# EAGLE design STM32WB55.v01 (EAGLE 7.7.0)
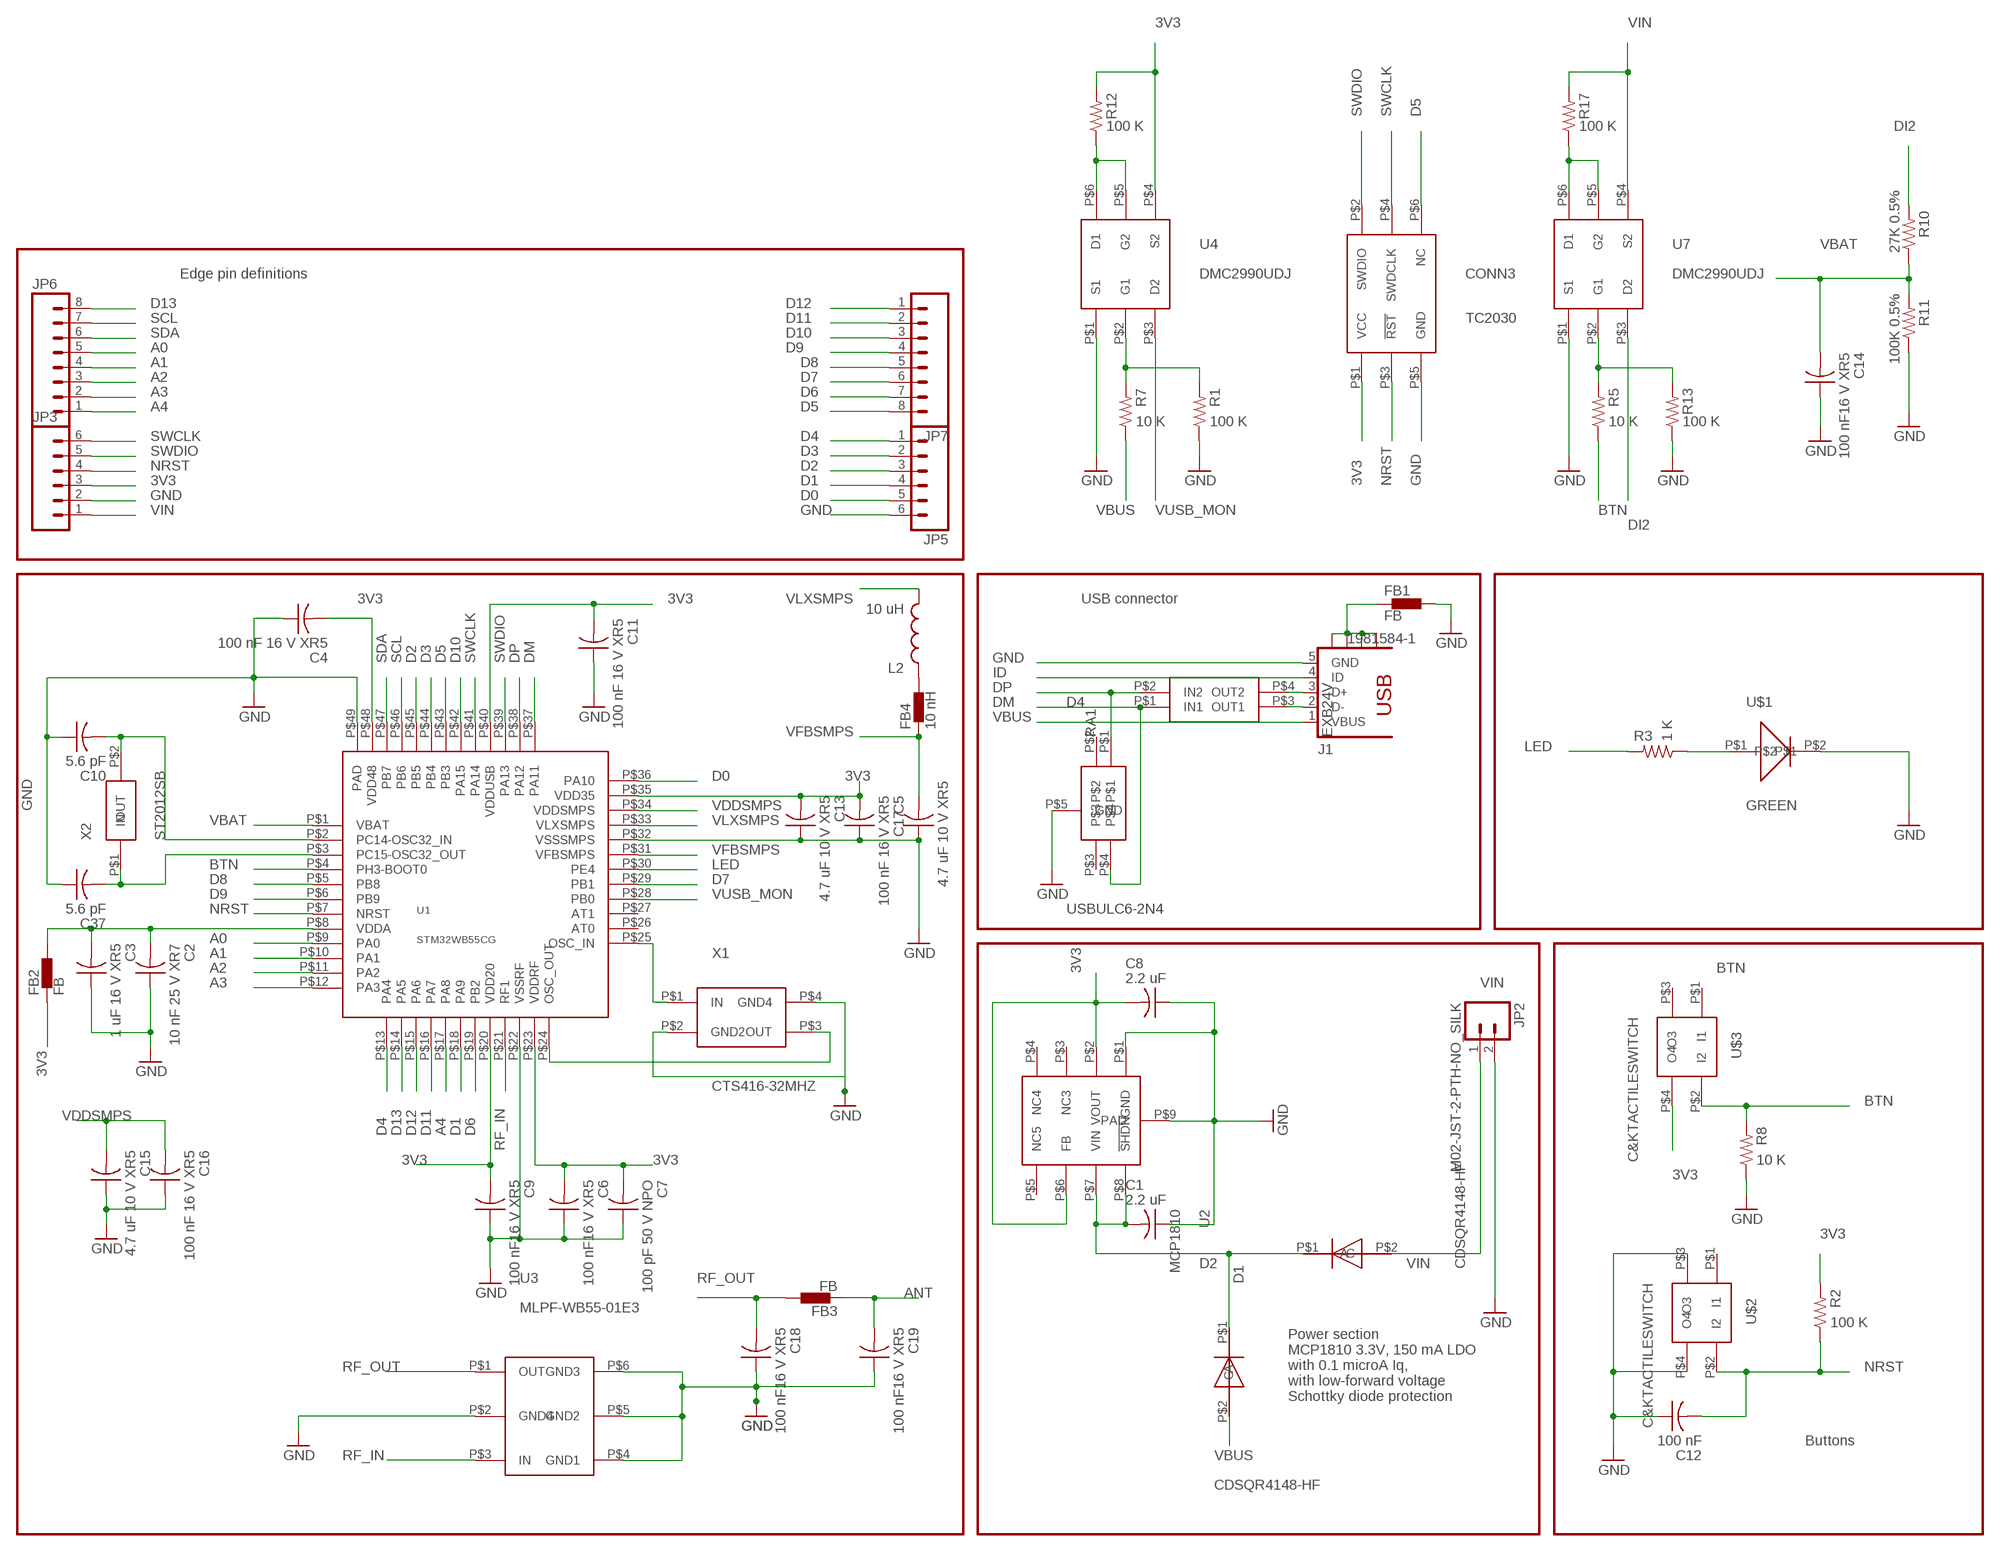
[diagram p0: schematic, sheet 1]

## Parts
C1  2.2 uF  C-US  [C0402_B]
C2  10 nF 25 V XR7  C-US  [C0402_B]
C3  1 uF 16 V XR5  C-US  [C0402_B]
C4  100 nF 16 V XR5  C-US  [C0402_B]
C5  100 nF 16 V XR5  C-US  [C0402_B]
C6  100 nF16 V XR5  C-US  [C0402_B]
C7  100 pF 50 V NPO  C-US  [C0402_B]
C8  2.2 uF  C-US  [C0402_B]
C9  100 nF16 V XR5  C-US  [C0402_B]
C10  5.6 pF  C-US  [C0402_B]
C11  100 nF 16 V XR5  C-US  [C0402_B]
C12  100 nF  C-US  [C0402_B]
C13  4.7 uF 10 V XR5  C-US  [C0402_B]
C14  100 nF16 V XR5  C-US  [C0402_B]
C15  4.7 uF 10 V XR5  C-US  [C0402_B]
C16  100 nF 16 V XR5  C-US  [C0402_B]
C17  4.7 uF 10 V XR5  C-US  [C0402_B]
C18  100 nF16 V XR5  C-US  [C0402_B]
C19  100 nF16 V XR5  C-US  [C0402_B]
C37  5.6 pF  C-US  [C0402_B]
CONN3  TC2030  [TC2030]
D1  CDSQR4148-HF  [CDSQR4148-HF]
D2  CDSQR4148-HF  [CDSQR4148-HF]
D4  USBULC6-2N4  [USBULC6-2N4]
FB1  FB  BLM15H  [0402]
FB2  FB  BLM15H  [0402]
FB3  FB  BLM15H  [0402]
FB4  10 nH  BLM15H  [0402]
J1  1981584-1  [1981584-1]
JP2  M02-JST-2-PTH-NO_SILK  [JST-2-PTH-NS]
JP3  M06NO_SILK  [1X06_NO_SILK]
JP5  M06NO_SILK  [1X06_NO_SILK]
JP6  M08NO_SILK  [1X08_NO_SILK]
JP7  M08NO_SILK  [1X08_NO_SILK]
L2  10 uH  INDUCTOR0805  [0805]
R1  100 K  R-US_  [R0402_B]
R2  100 K  R-US_  [R0402_B]
R3  1 K  R-US_  [R0402_B]
R5  10 K  R-US_  [R0402_B]
R7  10 K  R-US_  [R0402_B]
R8  10 K  R-US_  [R0402_B]
R10  27K 0.5%  R-US_  [R0402_B]
R11  100K 0.5%  R-US_  [R0402_B]
R12  100 K  R-US_  [R0402_B]
R13  100 K  R-US_  [R0402_B]
R17  100 K  R-US_  [R0402_B]
RA1  EXB24V  [EXB24V]
U1  STM32WB55CG  [ST32WB55CG]
U2  MCP1810  [MCP1810]
U3  MLPF-WB55-01E3  [MLPF-WB55-01E3]
U4  DMC2990UDJ  [DMC2990UDJ]
U7  DMC2990UDJ  [DMC2990UDJ]
U$1  GREEN  0402LED  [0402LED]
U$2  C&KTACTILESWITCH  [C&KTACTILESWITCH]
U$3  C&KTACTILESWITCH  [C&KTACTILESWITCH]
X1  CTS416-32MHZ  [CTS416-32MHZ]
X2  ST2012SB  [ST2012SB]

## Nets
3V3: C4.2 C5.2 C6.2 C7.2 C8.2 C9.2 C11.2 C13.2 CONN3.P$1(VCC) FB2.1 JP3.3 R2.2 R12.2 U1.P$20(VDD20) U1.P$23(VDDRF) U1.P$35(VDD35) U1.P$40(VDDUSB) U1.P$48(VDD48) U2.P$2(VOUT) U2.P$6(FB) U4.P$4(S2) U$3.P$4(O4)
A0: JP6.5 U1.P$9(PA0)
A1: JP6.4 U1.P$10(PA1)
A2: JP6.3 U1.P$11(PA2)
A3: JP6.2 U1.P$12(PA3)
A4: JP6.1 U1.P$17(PA8)
ANT: C19.2 FB3.1
BTN: R5.1 R8.2 U1.P$4(PH3-BOOT0) U$3.P$2(I2)
D0: JP5.5 U1.P$36(PA10)
D1: JP5.4 U1.P$18(PA9)
D2: JP5.3 U1.P$45(PB5)
D3: JP5.2 U1.P$44(PB4)
D4: JP5.1 U1.P$13(PA4)
D5: CONN3.P$6(NC) JP7.8 U1.P$43(PB3)
D6: JP7.7 U1.P$19(PB2)
D7: JP7.6 U1.P$29(PB1)
D8: JP7.5 U1.P$5(PB8)
D9: JP7.4 U1.P$6(PB9)
D10: JP7.3 U1.P$42(PA15)
D11: JP7.2 U1.P$16(PA7)
D12: JP7.1 U1.P$15(PA6)
D13: JP6.8 U1.P$14(PA5)
DI2: R10.2 U7.P$3(D2)
DM: D4.P$4 RA1.P$1(IN1) U1.P$37(PA11)
DP: D4.P$1 RA1.P$2(IN2) U1.P$38(PA12)
GND: C1.1 C2.1 C3.1 C4.1 C5.1 C6.1 C7.1 C8.1 C9.1 C10.1 C11.1 C12.1 C13.1 C14.1 C15.1 C16.1 C17.1 C18.1 C19.1 C37.1 CONN3.P$5(GND) D4.P$5(GND) FB1.2 J1.5(GND) JP2.2 JP3.2 JP5.6 R1.1 R8.1 R11.1 R13.1 U1.P$22(VSSRF) U1.P$32(VSSSMPS) U1.P$49(PAD) U2.P$1(GND) U2.P$9(PAD) U3.P$2(GND4) U3.P$4(GND1) U3.P$5(GND2) U3.P$6(GND3) U4.P$1(S1) U7.P$1(S1) U$1.P$2 U$2.P$3(O3) U$2.P$4(O4) X1.P$2(GND2) X1.P$4(GND4)
ID: J1.4(ID)
LED: R3.2 U1.P$30(PE4)
N$1: R3.1 U$1.P$1
N$2: C2.2 C3.2 FB2.2 U1.P$8(VDDA)
N$3: U1.P$25(OSC_IN) X1.P$1(IN)
N$4: U1.P$24(OSC_OUT) X1.P$3(OUT)
N$5: FB4.2 L2.1
N$7: C10.2 U1.P$2(PC14-OSC32_IN) X2.P$2(OUT)
N$8: C37.2 U1.P$3(PC15-OSC32_OUT) X2.P$1(IN)
N$10: R1.2 R7.2 U4.P$2(G1)
N$11: R12.1 U4.P$5(G2) U4.P$6(D1)
N$12: R5.2 R13.2 U7.P$2(G1)
N$13: R17.1 U7.P$5(G2) U7.P$6(D1)
N$31: J1.3(D+) RA1.P$4(OUT2)
N$33: J1.2(D-) RA1.P$3(OUT1)
NRST: C12.2 CONN3.P$3(!RST) JP3.4 R2.1 U1.P$7(NRST) U$2.P$2(I2)
PWRIN: C1.2 D1.P$1(C) D2.P$1(C) U2.P$7(VIN) U2.P$8(!SHDN)
RF_IN: U1.P$21(RF1) U3.P$3(IN)
RF_OUT: C18.2 FB3.2 U3.P$1(OUT)
SCL: JP6.7 U1.P$46(PB6)
SDA: JP6.6 U1.P$47(PB7)
SWCLK: CONN3.P$4(SWDCLK) JP3.6 U1.P$41(PA14)
SWDIO: CONN3.P$2(SWDIO) JP3.5 U1.P$39(PA13)
USB_SHIELD: FB1.1 J1.S1 J1.S2 J1.S3 J1.S4
VBAT: C14.2 R10.1 R11.2 U1.P$1(VBAT)
VBUS: D2.P$2(A) J1.1(VBUS) R7.1
VDDSMPS: C15.2 C16.2 U1.P$34(VDDSMPS)
VFBSMPS: C17.2 FB4.1 U1.P$31(VFBSMPS)
VIN: D1.P$2(A) JP2.1 JP3.1 R17.2 U7.P$4(S2)
VLXSMPS: L2.2 U1.P$33(VLXSMPS)
VUSB_MON: U1.P$28(PB0) U4.P$3(D2)
Unconnected: D4.P$2 D4.P$3 U1.P$26(AT0) U1.P$27(AT1) U2.P$3(NC3) U2.P$4(NC4) U2.P$5(NC5) U$2.P$1(I1) U$3.P$1(I1) U$3.P$3(O3)

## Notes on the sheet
- Edge pin definitions
- USB connector
- Power section
  MCP1810 3.3V, 150 mA LDO
  with 0.1 microA Iq, 
  with low-forward voltage 
  Schottky diode protection
- Buttons

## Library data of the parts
C1-C19 C37 = Spark:C-US: Capacitor
CONN3 = Kris:TC2030: TC2030 SWD pogo pin contact pad
D1 D2 = Kris:CDSQR4148-HF: ComChip's CDSQR4148-HF high speed 150 mA Io diode
D4 = Kris:USBULC6-2N4: ST TVS diode ESD Protection USBULC6-2N4
FB1-FB4 = STM32L433SARA.AssetTracker.v01:BLM15H: EMIFIL (R) Chip Ferrite Bead for GHz Noise
J1 = con-usb:1981584-1: Receptacle, micro-USB, type A/B Tyco Electronics; MF: Hirose; MPN: ZX62-AB-5PA(11)
JP2 = SparkFun-Connectors:M02: Standard 2-pin 0.1" header. Use with
JP3 JP5 = SparkFun-Connectors:M06: Header 6 Standard 6-pin 0.1" header. Use with straight break away headers (SKU : PRT-00116), right angle break away headers (PRT-00553), swiss pins (PRT-00743), machine pins (PRT-00117), and female headers (PRT-00115). Molex polarized connector foot print use with SKU : PRT-08094 with associated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
JP6 JP7 = SparkFun-Connectors:M08: Header 8 Standard 8-pin 0.1" header. Use with straight break away headers (SKU : PRT-00116), right angle break away headers (PRT-00553), swiss pins (PRT-00743), machine pins (PRT-00117), and female headers (PRT-00115).
L2 = SparkFun-Passives:INDUCTOR: Inductors
R1-R3 R5 R7 R8 R10-R13 R17 = Spark:R-US_: 0402 Resistor
RA1 = Kris:EXB24V: Panasonic EXB24 22 Ohm series resistor pair
U1 = Kris:STM32WB55CG: STM32WB55CG 7 mm x 7 mm UFQFPN48 https://www.st.com/en/microcontrollers/stm32wbx5.html?querycriteria=productId=LN2047
U2 = Kris:MCP1810: MCP1810 3.0 V Low Iq LDO http://ww1.microchip.com/downloads/en/DeviceDoc/20005623A.pdf
U3 = Kris:MLPF-WB55-01E3: MLPF-WB55-01E3
U4 U7 = Kris:DMC2990UDJ: DMC2990UDJ dual N-Type and P-Type MOSFET COMPLEMENTARY PAIR ENHANCEMENT MODE MOSFET https://www.diodes.com/assets/Datasheets/DMC2990UDJ.pdf
U$1 = Kris:0402LED: 0402led
U$2 U$3 = Kris:C&KTACTILESWITCH: C&K Tactile Switch 611-PTS810SJS250SMTR
X1 = Kris:CTS416-32MHZ: 32 MHz CTS416 crystal
X2 = Kris:ST2012SB: Kyocera 2.0 x 1.2 mm 32.768 20kHz ppm 4 pf crystal

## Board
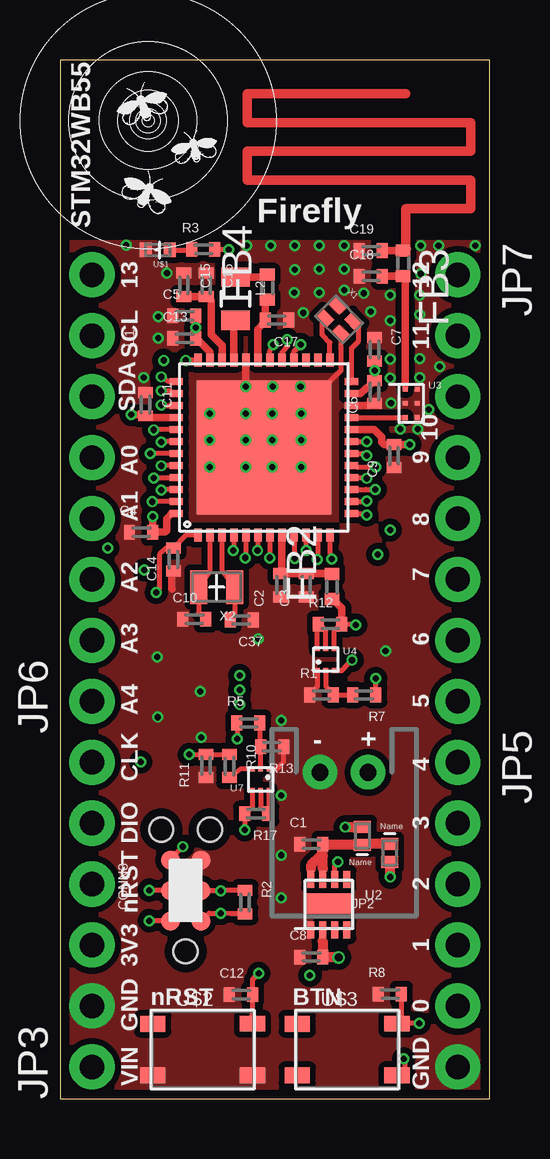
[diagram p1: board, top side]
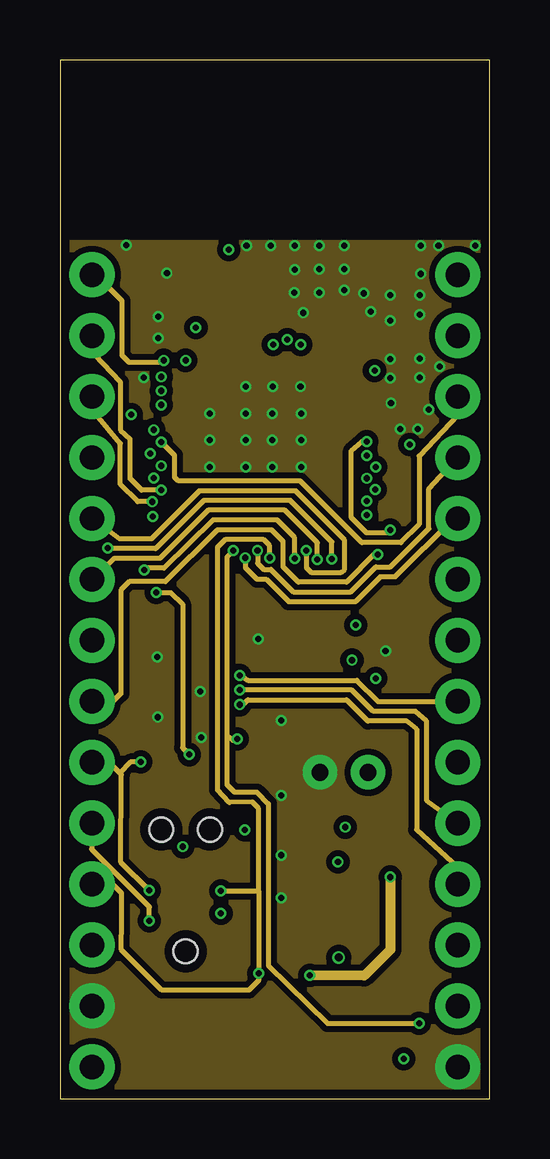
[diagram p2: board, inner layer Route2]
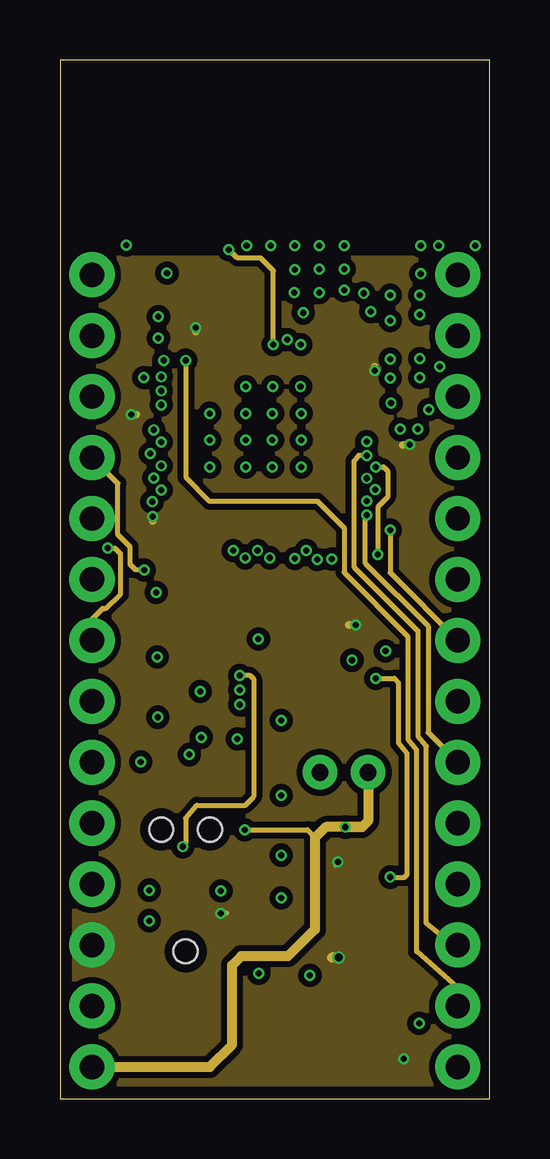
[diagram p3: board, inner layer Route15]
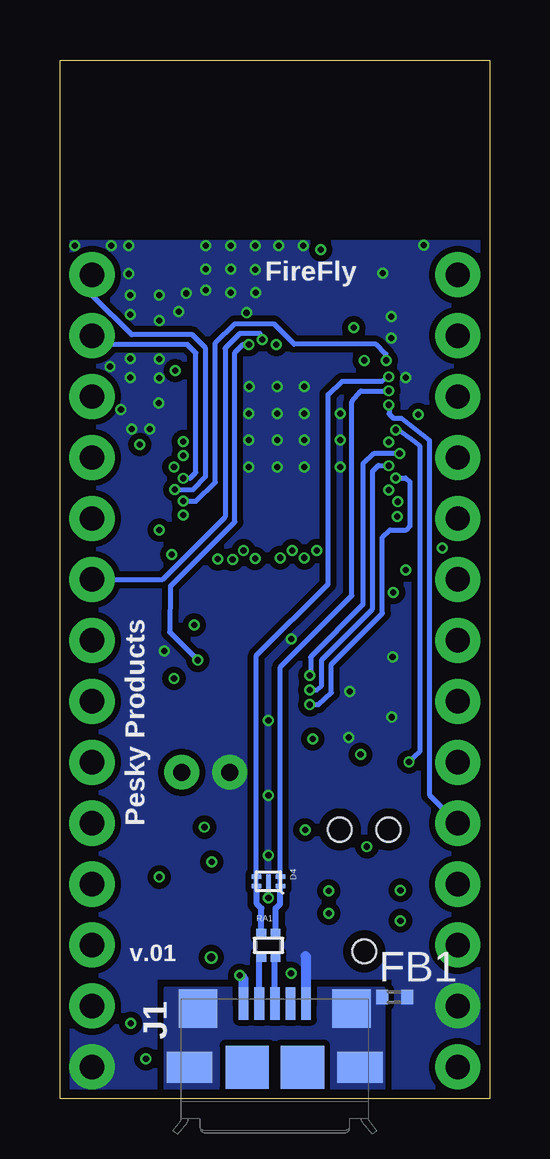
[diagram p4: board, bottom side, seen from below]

Size 17.91 x 43.31 mm. Coordinates in mm from the lower left corner, seen from the top.
Outline: 0,0 17.91,0 17.91,43.31 0,43.31 0,0
Copper layers (1*2*15*16): Top 0.035559375mm / dielectric 0.17018125mm / Route2 0.01778125mm / dielectric 47mil / Route15 0.01778125mm / dielectric 0.17018125mm / Bottom 0.035559375mm
Design rules "OSHPark-4layer *": minimum track width 5mil, minimum drill 10mil, track to track 5mil, track to pad 5mil, pad to pad 5mil, via to via 5mil, smd to smd 5mil, copper to edge 15mil, drill to drill 6mil, minimum pad ring 4mil, minimum via ring 4mil, stop-mask expansion 4mil, vias tented up to drill 20mil, thermal gap 10mil

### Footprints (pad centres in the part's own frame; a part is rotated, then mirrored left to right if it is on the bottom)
C0402_B = smd 0.457 x 0.61: 1 -0.483,0; 2 0.483,0
TC2030 = smd 0.787 x 0.787: P$1 -1.27,-0.635; P$2 -1.27,0.635; P$3 0,-0.635; P$4 0,0.635; P$5 1.27,-0.635; P$6 1.27,0.635 | hole 0.991: -2.54,0; 2.54,1.016; 2.54,-1.016
CDSQR4148-HF = smd 0.7 x 0.5: P$1 0,0.375; P$2 0,-0.375
USBULC6-2N4 = smd 0.2 x 0.4: P$1 0.2,0.5; P$2 -0.2,0.5; P$3 -0.2,-0.5; P$4 0.2,-0.5 | smd 0.6 x 0.2: P$5 0,0
0402 = smd 0.5 x 0.61: 1 -0.5,0; 2 0.55,0
1981584-1 = smd 0.4 x 1.35: 1 -1.3,4.1; 2 -0.65,4.1; 3 0,4.1; 4 0.65,4.1; 5 1.3,4.1 | smd 1.8 x 1.8: M1 -1.15,1.45; M2 1.15,1.45 | smd 1.9 x 1.3: S1 -3.55,1.45; S2 3.55,1.45 | smd 1.6 x 1.6: S3 -3.2,3.885; S4 3.2,3.885
JST-2-PTH-NS = drill 0.7 pad 1.448: 1 -1,0; 2 1,0
1X06_NO_SILK = drill 1.016 pad 1.88: 1 0,0; 2 2.54,0; 3 5.08,0; 4 7.62,0; 5 10.16,0; 6 12.7,0
1X08_NO_SILK = drill 1.016 pad 1.88: 1 0,0; 2 2.54,0; 3 5.08,0; 4 7.62,0; 5 10.16,0; 6 12.7,0; 7 15.24,0; 8 17.78,0
0805 = smd 0.8 x 1.2: 1 -0.9,0; 2 0.9,0
R0402_B = smd 0.457 x 0.61: 1 -0.483,0; 2 0.483,0
EXB24V = smd 0.4 x 0.36: P$1 -0.3,0.5; P$2 0.3,0.5; P$3 -0.3,-0.5; P$4 0.3,-0.5
ST32WB55CG = smd 0.55 x 0.3: P$1 -3.65,2.75; P$2 -3.65,2.25; P$3 -3.65,1.75; P$4 -3.65,1.25; P$5 -3.65,0.75; P$6 -3.65,0.25; P$7 -3.65,-0.25; P$8 -3.65,-0.75; P$9 -3.65,-1.25; P$10 -3.65,-1.75; P$11 -3.65,-2.25; P$12 -3.65,-2.75; P$25 3.65,-2.75; P$26 3.65,-2.25; P$27 3.65,-1.75; P$28 3.65,-1.25; P$29 3.65,-0.75; P$30 3.65,-0.25; P$31 3.65,0.25; P$32 3.65,0.75; P$33 3.65,1.25; P$34 3.65,1.75; P$35 3.65,2.25; P$36 3.65,2.75 | smd 0.3 x 0.55: P$13 -2.75,-3.65; P$14 -2.25,-3.65; P$15 -1.75,-3.65; P$16 -1.25,-3.65; P$17 -0.75,-3.65; P$18 -0.25,-3.65; P$19 0.25,-3.65; P$20 0.75,-3.65; P$21 1.25,-3.65; P$22 1.75,-3.65; P$23 2.25,-3.65; P$24 2.75,-3.65; P$37 2.75,3.65; P$38 2.25,3.65; P$39 1.75,3.65; P$40 1.25,3.65; P$41 0.75,3.65; P$42 0.25,3.65; P$43 -0.25,3.65; P$44 -0.75,3.65; P$45 -1.25,3.65; P$46 -1.75,3.65; P$47 -2.25,3.65; P$48 -2.75,3.65 | smd 5.6 x 5.6: P$49 0,0
MCP1810 = smd 0.3 x 0.7: P$1 -0.75,-1.05; P$2 -0.25,-1.05; P$3 0.25,-1.05; P$4 0.75,-1.05; P$5 0.75,1.05; P$6 0.25,1.05; P$7 -0.25,1.05; P$8 -0.75,1.05 | smd 1.95 x 0.95: P$9 0,0
MLPF-WB55-01E3 = smd 0.2 x 0.2: P$1 -0.25,0.587; P$2 -0.25,0; P$3 -0.25,-0.587; P$4 0.25,-0.587; P$5 0.25,0; P$6 0.25,0.587
DMC2990UDJ = smd 0.2 x 0.2: P$1 -0.35,-0.45; P$2 0,-0.45; P$3 0.35,-0.45; P$4 0.35,0.45; P$5 0,0.45; P$6 -0.35,0.45
0402LED = smd 0.5 x 0.6: P$1 -0.5,0; P$2 0.5,0
C&KTACTILESWITCH = smd 1.05 x 0.65: P$1 -2.075,1.073; P$2 2.075,1.075; P$3 -2.075,-1.075; P$4 2.075,-1.075
CTS416-32MHZ = smd 0.67 x 0.48: P$1 -0.485,-0.38; P$2 0.485,-0.38; P$3 0.485,0.38; P$4 -0.485,0.38
ST2012SB = smd 0.7 x 1.4: P$1 -0.75,0; P$2 0.75,0

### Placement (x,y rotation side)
C1  10.46,10.62 0 top
C2  9.19,21.41 90 top
C3  10.26,21.41 90 top
C4  3.38,23.62 0 top
C5  5.18,32.64 0 top
C6  13.11,29.46 90 top
C7  13.11,31.24 270 top
C8  10.46,5.92 0 top
C9  13.92,26.8 90 top
C10  5.59,19.99 0 top
C11  3.56,28.96 270 top
C12  7.54,4.34 0 top
C13  5.18,31.7 0 top
C14  4.72,22.48 90 top
C15  5.16,33.93 270 top
C16  6.1,33.93 270 top
C17  9.04,32.46 180 top
C18  12.95,34.29 0 top
C19  12.95,35.36 0 top
C37  7.57,19.96 180 top
CONN3  5.23,8.69 90 top
D1  12.6,10.97 180 top
D2  13.74,10.26 0 top
D4  9.22,9.07 270 bottom
FB1  3.99,4.24 0 bottom
FB2  11.33,21.34 90 top
FB3  14.3,34.85 270 top
FB4  8.64,33.81 90 top
J1  8.95,-0.13 0 bottom
JP2  11.84,13.61 180 top
JP3  1.33,1.33 90 top
JP5  16.57,14.03 270 top
JP6  1.33,16.57 90 top
JP7  16.57,34.35 270 top
L2  7.32,33.35 270 top
R1  10.9,16.84 0 top
R2  7.71,8.2 270 top
R3  5.97,35.41 0 top
R5  7.85,15.67 0 top
R7  12.67,16.84 180 top
R8  13.74,4.37 0 top
R10  7.06,13.88 270 top
R11  6.08,13.88 90 top
R12  11.25,19.79 0 top
R13  8.84,14.68 180 top
R17  8.18,11.89 180 top
RA1  9.22,6.4 0 bottom
U1  8.5,27.15 90 top
U2  11.2,8.1 0 top
U3  14.63,28.99 0 top
U4  11.07,18.31 0 top
U7  8.36,13.31 180 top
U$1  4.06,35.38 180 top
U$2  5.94,2.06 0 top
U$3  11.96,2.06 0 top
X1  11.63,32.49 315 top
X2  6.53,21.34 180 top

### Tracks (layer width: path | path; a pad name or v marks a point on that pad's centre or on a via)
3V3  (via drill 0.25, 0.33)
  Top 0.203: U2.P$6 11.45,9.72 v11.58,9.88 | U$3.P$4 14.38,1.22 14.38,1.63 v14.33,1.68 | U4.P$4 11.42,19.58 R12.2 12.27,19.79 v12.32,19.76 | CONN3.P$1 6.21,7.73 v6.71,7.73 7.1,7.72 R2.2
  Top 0.305: U1.P$35 6.25,31.14 5.69,31.7 5.69,31.67 C13.2 v5.66,32.16 C5.2 | U1.P$40 3.54,28.4 3.53,28.4 3.45,28.4 | C7.2 v13.11,30.35 C6.2 12.51,29.4 U1.P$23 | 10.95,5.87 C8.2 | U2.P$2 10.95,6.58 | v3.86,24.28 C4.2 4.37,23.62 4.45,23.7 4.45,24.18 4.64,24.4 U1.P$48 | v14.58,27.28 C9.2 13.51,27.28 13.41,27.38 13.41,27.58 13.09,27.9 U1.P$20 | 3.45,28.4 C11.2 3.33,28.5 v2.97,28.52 | 3.45,28.4 3.45,28.42 | FB2.1 11.37,20.84 11.73,20.47 R12.2
  Top 0.406: v11.61,5.89 11.53,5.92 C8.2 10.95,6.58
  Route15 0.203: v11.58,9.88 11.48,9.75 | v14.33,1.68 14.33,1.63 14.38,1.57 | v6.71,7.73 6.95,7.73
  Route15 0.305: v5.66,32.16 5.66,31.98 | v12.32,19.76 12.04,19.76 | v2.97,28.52 3.17,28.52 | v13.11,30.35 13.11,30.53 | v3.86,24.28 3.86,24.08 | v14.58,27.28 14.28,27.25
  Route15 0.406: v11.61,5.89 11.33,5.89
  pour Route15 (isolate 0.254, no thermals): 0.64,35.05 17.27,35.05 17.27,0.64 0.64,0.64
A0  (via drill 0.25)
  Top 0.203: v9.78,22.53 9.78,23.41 U1.P$9
  Route2 0.203: v9.78,22.53 9.78,23.39 9.04,24.13 6.38,24.13 4.34,22.12 3.5,22.12 v3.5,22.05
  Route15 0.203: v3.5,22.05 3.15,22.05 2.92,22.28 2.92,23.01 2.41,23.52 2.41,25.65 JP6.5
A1  (via drill 0.25)
  Top 0.203: U1.P$10 10.25,22.88 v10.26,22.86
  Route2 0.203: JP6.4 2.49,23.34 3.81,23.34 5.82,25.35 9.8,25.35 11.86,23.29 11.86,22.07 11.71,21.95 10.46,21.95 10.26,22.15 v10.26,22.86
A2  (via drill 0.25)
  Top 0.203: U1.P$11 10.75,22.58 v10.72,22.48
  Route2 0.203: v10.72,22.48 10.72,23.19 9.37,24.54 6.17,24.54 4.17,22.53 2.26,22.53 JP6.3
A3  (via drill 0.25)
  Top 0.203: U1.P$12 11.25,22.69 v11.33,22.5
  Route2 0.203: v11.33,22.5 11.33,23.22 9.6,24.94 5.99,24.94 3.99,22.94 2.08,22.94 v1.98,22.96
  Route15 0.203: v1.98,22.96 2.29,22.96 2.52,22.73 2.52,21.03 1.91,20.45 1.78,20.45 1.33,20 JP6.2
A4  (via drill 0.25)
  Top 0.203: U1.P$17 12.33,26.4 12.37,26.34 v13.16,26.34
  Route2 0.203: JP6.1 1.35,16.59 2.21,16.59 2.54,16.89 2.54,21.21 2.9,21.57 4.39,21.57 6.55,23.72 8.81,23.72 9.3,23.24 9.3,22.17 9.93,21.54 11.94,21.54 13.08,22.68 v13.25,22.7
  Route15 0.203: v13.25,22.7 13.25,24.66 13.65,25.09 13.65,26.18 13.49,26.34 v13.16,26.34
ANT
  Top 0.305: C19.2 14.22,35.36 FB3.1
  Top 0.4: 14.41,35.43 14.41,37.1 17.11,37.1 17.11,38.3 7.81,38.3 7.81,39.5 17.11,39.5 17.11,40.7 7.81,40.7 7.81,41.9 14.41,41.9
  Top 0.406: FB3.1 14.32,35.35 14.41,35.43
BTN  (via drill 0.25)
  Top 0.203: U1.P$4 7.25,22.94 v7.21,22.86 | v14.96,3.15 13.98,3.15 U$3.P$2 14.22,3.39 R8.2 | R5.1 v7.38,15
  Route2 0.203: v14.96,3.15 11.15,3.15 8.69,5.56 8.69,12.31 8.22,12.78 7.28,12.78 6.96,13.09 6.96,15.14 | 6.96,15.14 6.96,22.58 v7.21,22.86 | v7.38,15 7.19,14.95 6.96,15.14
D0  (via drill 0.25)
  Top 0.203: U1.P$36 5.33,30.8 v5.23,30.79
  Route15 0.203: JP5.5 16.57,4.64 14.86,6.15 14.86,14.55 14.5,14.99 14.5,19.25 11.84,21.95 11.84,23.8 10.72,24.92 6.22,24.92 5.26,25.91 5.26,30.76 v5.23,30.79
D1  (via drill 0.25)
  Top 0.203: U1.P$18 12.62,26.9 v12.78,26.81
  Route15 0.203: JP5.4 16.34,6.41 15.27,7.32 15.27,14.71 14.91,15.14 14.91,19.51 12.24,22.17 12.24,26.59 12.45,26.82 v12.78,26.81
D2  (via drill 0.25)
  Top 0.203: U1.P$45 4.7,25.9 4.67,25.93 4.7,25.93 4.62,25.88 v3.91,25.88
  Route2 0.203: JP5.3 16.59,8.97 16.59,9.65 14.86,11.23 14.86,15.42 14.45,15.75 12.83,15.75 11.94,16.64 7.82,16.64 7.64,16.43 v7.49,16.43
  Bottom 0.203: v3.91,25.88 3.5,25.88 3.33,25.73 3.33,23.88 3.48,23.72 4.17,23.72 4.47,23.42 4.47,20.24 6.6,18.11 6.6,16.94 7.14,16.43 v7.49,16.43
D3  (via drill 0.25)
  Top 0.203: U1.P$44 4.25,26.4 v4.22,26.39
  Route2 0.203: v7.49,17.04 12.17,17.04 13.06,16.15 14.81,16.15 15.27,15.75 15.27,12.45 JP5.2
  Bottom 0.203: v4.22,26.39 4.31,26.4 4.64,26.4 4.88,26.17 4.88,20.42 7.01,18.29 7.01,17.22 7.21,17.04 v7.49,17.04
D4  (via drill 0.25)
  Top 0.203: U1.P$13 12.68,24.4 v12.78,24.33
  Route15 0.203: JP5.1 15.34,15.27 15.34,19.71 12.72,22.33 12.72,24.16 v12.78,24.33
D5  (via drill 0.25)
  Top 0.203: U1.P$43 v3.76,26.9 | CONN3.P$6 4.6,10.03 v5.12,10.52
  Route2 0.203: JP7.8 13.26,16.56 12.37,17.45 7.82,17.45 7.57,17.65 v7.49,17.65
  Route15 0.203: 7.48,17.67 7.52,17.67 | 7.52,17.67 7.9,17.67 8.06,17.5 8.06,12.6 7.71,12.24 5.7,12.24 5.23,11.7 5.23,10.63 v5.12,10.52 | v7.49,17.65 7.51,17.65 7.52,17.67
  Bottom 0.203: v3.76,26.9 4.83,26.9 5.28,26.47 5.28,20.6 7.47,18.41 7.47,17.7 v7.49,17.65
D6  (via drill 0.25)
  Top 0.203: U1.P$19 12.72,27.4 v12.78,27.39
  Route2 0.203: v13.77,23.71 13.6,23.6 12.78,23.6 12.14,24.23 12.14,27.03 12.57,27.41 12.76,27.41 v12.78,27.39
  Route15 0.203: v13.77,23.71 13.75,21.93 JP7.7
D7  (via drill 0.25)
  Top 0.203: U1.P$29 9.25,31.09 9.47,31.37 v9.47,31.65
  Bottom 0.203: v9.47,31.65 9.47,31.77 9.58,31.9 10.41,31.9 11.02,31.29 11.02,24.26 13.63,21.65 JP7.6
D8  (via drill 0.25)
  Top 0.203: U1.P$5 7.75,22.61 v7.72,22.55
  Route2 0.203: v7.72,22.55 7.72,22.15 8.2,21.67 8.59,21.67 9.53,20.73 12.32,20.73 13.36,21.77 13.97,21.77 16.38,24.18 JP7.5
D9  (via drill 0.25)
  Top 0.203: U1.P$6 8.25,22.98 v8.23,22.86
  Route2 0.203: JP7.4 15.37,25.43 15.37,23.77 13.77,22.17 13.16,22.17 12.12,21.13 9.73,21.13 8.79,22.07 8.48,22.07 8.23,22.33 v8.23,22.86
D10  (via drill 0.25)
  Top 0.203: U1.P$42 4.42,27.4 v4.22,27.38
  Route2 0.203: JP7.3 16.57,28.51 14.96,26.8 14.96,23.95 14.2,23.19 12.57,23.19 10.01,25.76 4.93,25.76 4.78,25.91 4.78,26.82 v4.22,27.38
D11  (via drill 0.25)
  Top 0.203: U1.P$16 12.71,25.9 v12.78,25.87
  Bottom 0.203: v12.78,25.87 12.48,25.87 12.24,26.11 12.24,31.09 12.6,31.45 16.15,31.45 JP7.2
D12  (via drill 0.25)
  Top 0.203: U1.P$15 12.75,25.4 v13.13,25.4
  Bottom 0.203: v13.13,25.4 12.36,25.4 11.84,25.93 11.84,31.29 12.39,31.85 14.91,31.85 16.57,33.49 JP7.1
D13  (via drill 0.25)
  Top 0.203: U1.P$14 12.66,24.9 v12.78,24.92
  Route2 0.203: JP6.8 1.5,34.35 2.58,33.27 2.58,31 2.87,30.71 4.24,30.71 v4.32,30.79
  Bottom 0.203: v12.78,24.92 12.24,24.92 11.43,25.7 11.43,31.52 10.62,32.31 9,32.31 8.15,31.46 4.74,31.46 4.33,31.05 4.33,30.79 v4.32,30.79
DI2
  Top 0.203: U7.P$3 7.54,13.76 R10.2
DM  (via drill 0.25)
  Top 0.203: U1.P$37 4.51,29.9 v4.22,30.1
  Bottom 0.203: D4.P$4 9.72,18.47 6.73,21.46 6.73,29.36 6.15,29.92 4.48,29.92 v4.22,30.1
  Bottom 0.254: RA1.P$1 9.52,7.95 9.7,8.13 9.7,8.85 D4.P$4
DP  (via drill 0.25)
  Top 0.203: U1.P$38 4.56,29.52 v4.22,29.52
  Bottom 0.203: D4.P$1 8.72,18 5.74,20.98 5.74,29.06 5.37,29.52 v4.22,29.52
  Bottom 0.254: RA1.P$2 8.92,7.95 8.74,8.13 8.74,8.85 D4.P$1
GND  (via drill 0.25)
  Top 0.203: X1.P$2 11.71,30.35 v8.85,27.46 | U4.P$1 10.72,17.2 R1.1 | U7.P$1 9.06,13.76 9.32,14.05 R13.1
  Top 0.305: U1.P$32 7.75,29.95 7.75,30.02 | U1.P$22 13.08,28.9 C6.1 | C14.1 4.65,22.05 4.65,21.29 4.67,21.26
  Bottom 0.203: D4.P$5 v9.22,8.38
  Bottom 0.406: J1.5 7.65,5.93 7.67,5.94
  other vias: 7.73,27.46 11.84,35.56 15.04,35.56 14.99,33.5 13.77,33.5 12.65,33.58 13.77,32.44 14.99,32.69 13.77,30.84 14.99,30.86 14.99,30.07 13.77,30.05 13.79,29.01 9.22,10.16 9.22,12.65 6.24,28.57 8.85,26.34 7.73,29.69 8.85,28.57 7.73,28.57 7.73,26.34 6.24,26.34 6.24,27.46 12.95,32.82 2.76,35.59 4.46,34.42 4.1,32.6 15.37,28.73 15.82,30.53 14.91,27.91 10.79,35.56 9.78,35.56 8.79,35.56 7.77,35.56 11.84,34.59 10.79,34.59 11.84,33.71 17.3,35.56 15.77,35.56 15.04,34.39 10.05,28.57 10.05,27.46 10.05,26.34 8.27,19.18 9.22,15.77 13.56,18.67 3.49,30.06 4.1,31.71 9.78,34.57 10.79,33.6 9.75,33.6 10.13,32.77 14.17,27.91 4.05,18.43 4.08,15.91 5.84,16.98 5.88,15.07 10.02,29.69 8.86,29.69
  pour Route2 (isolate 0.254, no thermals): 0,35.69 17.91,35.69 17.91,0 0,0
  pour Top (isolate 0.254, no thermals): 0,35.69 17.91,35.69 17.91,0 0,0
  pour Bottom (isolate 0.254, no thermals): 13.97,0 17.91,0 17.91,35.69 0,35.69 0,0 3.96,0 3.96,5.08 13.97,5.08
LED  (via drill 0.25)
  Top 0.203: U1.P$30 8.75,31.2 v8.89,31.45 | v7.04,35.41 R3.2
  Route15 0.203: v8.89,31.45 8.89,34.52 8.36,35.05 7.39,35.05 v7.04,35.41
N$1
  Top 0.203: U$1.P$1 5.46,35.38 R3.1
N$2
  Top 0.305: U1.P$8 9.25,21.95 C2.2 C3.2 FB2.2
N$3
  Top 0.203: U1.P$25 11.25,31.53 10.92,31.85 10.92,32.54 X1.P$1
N$4
  Top 0.203: U1.P$24 12.15,31.3 12.45,31.6 12.45,32.29 X1.P$3
N$5
  Top 0.305: L2.1 8.52,34.25 FB4.2
N$7
  Top 0.203: U1.P$2 6.25,21.96 X2.P$2 5.78,20.28 C10.2
N$8
  Top 0.203: U1.P$3 6.75,22.02 X2.P$1 7.28,20.21 C37.2
N$10
  Top 0.203: U4.P$2 11.07,17.2 R1.2 R7.2
N$11
  Top 0.203: U4.P$5 11.07,19.56 R12.1 10.72,19.79 U4.P$6
N$12
  Top 0.203: U7.P$2 R13.2 | 8.33,14.76 R13.2 | R5.2 8.33,14.71 R13.2
N$13
  Top 0.203: U7.P$5 8.36,12.14 R17.1 8.71,11.79 U7.P$6
N$31
  Bottom 0.254: J1.3 8.95,5.87 RA1.P$4
N$33
  Bottom 0.254: J1.2 9.6,5.82 RA1.P$3
NRST  (via drill 0.25)
  Top 0.203: U$2.P$2 C12.2 8.03,4.98 v8.28,5.23 | U1.P$7 8.75,22.67 v8.74,22.55 | CONN3.P$3 6.69,8.69 v6.71,8.67 6.72,8.69 R2.1
  Route2 0.203: v8.74,22.55 8.74,23.06 8.48,23.32 6.88,23.32 6.55,22.99 6.55,12.89 7.06,12.36 8.01,12.37 8.28,12.1 8.28,8.67 | 8.28,8.67 v8.28,5.23 | 8.27,5.22 v8.28,5.23 | v6.71,8.67 8.28,8.67 | v8.28,5.23 8.28,4.94 7.87,4.53 4.24,4.53 2.55,6.22 2.56,7.49 2.56,8.57 2.2,8.94 1.35,8.94 JP3.4
PWRIN
  Top 0.305: U2.P$7 10.95,9.6 | 10.45,9.6 U2.P$8
  Top 0.406: D2.P$1 12.97,10.64 D1.P$1 11.02,10.6 C1.2 10.95,10.11 | 10.95,9.6 10.95,10.11 | 10.45,9.6 10.45,9.73 10.88,10.16 10.95,10.11
RF_IN
  Top 0.203: U1.P$21 U3.P$3
RF_OUT
  Top 0.203: U3.P$1 14.38,29.57 14.38,29.77
  Top 0.305: C18.2 14.21,34.29 FB3.2 14.38,34.15 14.38,29.77
SCL  (via drill 0.25)
  Top 0.203: U1.P$46 4.24,25.4 v4.22,25.38
  Route2 0.203: JP6.7 1.44,31.71 1.44,31.03 2.52,29.87 2.52,27.89 2.92,27.51 2.92,25.86 3.4,25.38 v4.22,25.38
SDA  (via drill 0.25)
  Top 0.203: U1.P$47 3.83,24.9 v3.83,24.89
  Route2 0.203: v3.83,24.89 3.23,24.89 2.52,25.61 2.52,27.33 1.52,28.52 1.52,29.09 JP6.6
SWCLK  (via drill 0.25)
  Top 0.203: 4.81,27.94 U1.P$41 4.08,27.9 v3.91,27.89 | CONN3.P$4 3.68,8.69 v3.72,8.7
  Route2 0.203: v3.72,8.7 3.71,8.69 2.54,9.87 2.55,13.53 2.48,13.6 | 2.48,13.6 2.03,14.05 1.35,14.05 JP3.6 | v3.37,14.05 2.93,14.05 2.48,13.6
  Bottom 0.203: v3.91,27.89 3.79,27.89 3.28,27.51 2.92,27.23 2.92,14.46 v3.37,14.05
SWDIO  (via drill 0.25)
  Top 0.203: v4.22,28.93 4.29,28.91 U1.P$39 | CONN3.P$2 3.73,7.42 v3.72,7.43
  Route2 0.203: JP3.5 1.32,10.4 3.72,8 v3.72,7.43
  Bottom 0.203: JP3.5 2.52,12.68 2.52,27.46 3.68,28.37 4.01,28.37 4.19,28.55 4.19,28.88 v4.22,28.93
USB_SHIELD
  pour Bottom (isolate 0.254, no thermals): 4.47,0 13.46,0 13.46,4.57 4.47,4.57
VBAT  (via drill 0.25)
  Top 0.203: U1.P$1 5.24,23.5 C14.2 4.42,22.96 4.14,22.68 4.14,21.26 v4.01,21.11 | R10.1 R11.2 v5.38,14.35
  Route2 0.203: v4.01,21.11 4.62,21.11 5.11,20.62 5.11,14.63 v5.38,14.35
VBUS  (via drill 0.25)
  Top 0.203: R7.1 v13.16,17.53
  Top 0.406: v13.77,9.25 13.77,9.86 D2.P$2
  Route2 0.406: v13.77,9.25 13.77,6.22 12.68,5.13 v10.41,5.16
  Route15 0.203: 13.72,9.3 v13.77,9.25 13.79,9.22 14.33,9.22 14.45,9.35 14.45,14.4 14.1,14.83 14.1,17.35 13.95,17.53 v13.16,17.53
  Bottom 0.406: J1.1 10.25,5 v10.41,5.16
VDDSMPS
  Top 0.305: C15.2 C16.2 6.12,33.4 6.3,33.27 6.3,31.85 6.76,31.39 6.76,30.81 U1.P$34
VFBSMPS
  Top 0.305: U1.P$31 8.25,32.07 C17.2 8.56,33.23 FB4.1
VIN  (via drill 0.25)
  Top 0.203: U7.P$4 8.01,12.12 R17.2 v7.7,11.21
  Top 0.406: v11.89,11.33 12.41,11.33 D1.P$2
  Route15 0.203: v7.7,11.21 10.31,11.21 10.62,10.87
  Route15 0.406: JP2.1 12.84,11.59 D1.P$2 | D1.P$2 11.91,11.35 v11.89,11.33 | v11.89,11.33 12.58,11.33 D1.P$2 | JP3.1 6.25,1.33 7.18,2.26 7.18,5.58 7.54,5.94 9.5,5.94 10.62,7.06 10.62,10.87 11.07,11.33 v11.89,11.33
VLXSMPS
  Top 0.203: 7.2,32.68 L2.2
  Top 0.305: U1.P$33 7.25,32.49 L2.2
VUSB_MON  (via drill 0.25)
  Top 0.203: U4.P$3 11.77,17.86 v12.17,18.29 | U1.P$28 9.75,31.16 v10.03,31.45
  Bottom 0.203: v10.03,31.45 10.29,31.45 10.62,31.11 10.62,24.05 13.31,21.36 13.34,19.46 v12.17,18.29

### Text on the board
tPlace: Firefly | STM32WB55 | 13 | 12 | SCL | 11 | SDA | 10 | A0 | 9 | A1 | 8 | 7 | A2 | A3 | 6 | A4 | 5 | - | + | 4 | CLK | DIO | 3 | 2 | nRST | 3V3 | 1 | nRST | BTN | 0 | GND | VIN | GND
bPlace: FireFly | Pesky Products | v.01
